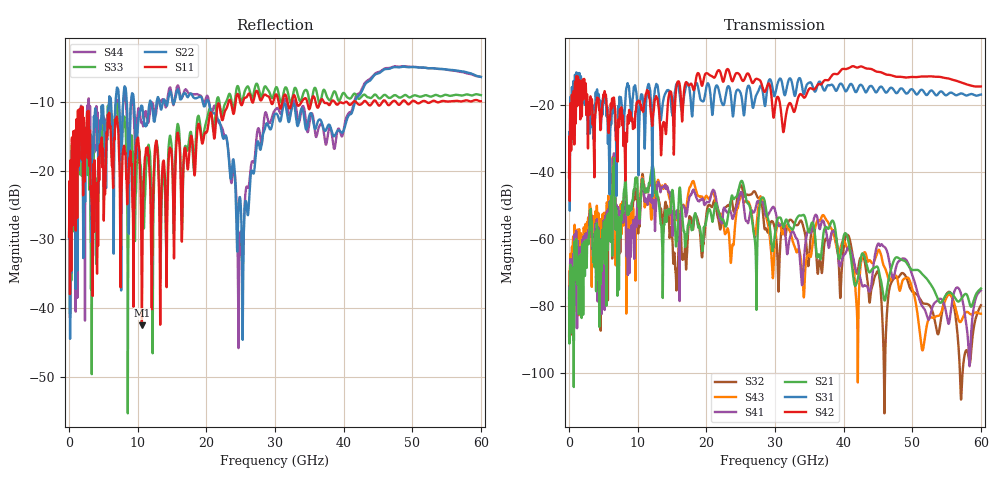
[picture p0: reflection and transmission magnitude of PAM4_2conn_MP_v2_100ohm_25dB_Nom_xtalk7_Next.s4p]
! Info: Touchstone file created by Circ.  Input file=FAB50GbE_2conn_Midplane_Examax_Topo2_v2_100ohm_25dB_Nom.circ
# Hz S RI R 50
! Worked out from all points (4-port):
!   6000 points, 10 MHz to 60 GHz, reference 50 ohm
!   strongest paths, dB at 10 MHz, 15.01 GHz, 30.01 GHz, 45.01 GHz, 60 GHz:
!     S42: -41.7, -18.2, -20.8, -10.2, -14.6
!     S31: -41.6, -22.6, -17.0, -15.7, -17.0
!     S21: -75.8, -45.7, -58.2, -68.7, -74.9
!     S41: -89.1, -56.3, -51.5, -61.6, -75.4
!     S43: -77.6, -54.9, -60.7, -63.6, -82.4
!     S32: -81.0, -59.0, -57.3, -69.8, -79.9
!   lowest |S11| = -42.5 dB at 10.61 GHz (marker M1), VSWR 1.02, Z = 49.5 + j0.506 ohm
!   |S11| at or under -10 dB: start of sweep to 23.25 GHz; 38.68 GHz to 40.3 GHz (1.616 GHz wide, 4.09 % of centre); 41.79 GHz to 42.9 GHz (1.107 GHz wide, 2.62 % of centre)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
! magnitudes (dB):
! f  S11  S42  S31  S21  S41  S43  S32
! 10 MHz  -29.6  -41.7  -41.6  -75.8  -89.1  -77.6  -81.0
! 1.29 GHz  -11.2  -11.7  -10.6  -65.6  -61.5  -60.0  -63.0
! 10.61 GHz  -42.5  -21.4  -16.9  -43.1  -42.9  -42.0  -41.8
! 15.61 GHz  -16.5  -15.2  -14.0  -61.8  -53.8  -54.4  -73.6
! 24.87 GHz  -9.7  -11.1  -16.0  -43.9  -46.9  -48.0  -44.5
! 28.66 GHz  -9.0  -15.7  -19.2  -50.8  -53.2  -53.3  -57.0
! 60 GHz  -9.9  -14.6  -17.0  -74.9  -75.4  -82.4  -79.9
